PROGRAM DwordToByteArray  //Convert integer value to byte array
VAR_INPUT 
	diValue : DINT;
	Datalenght : DWORD ; 
END_VAR
VAR_IN_OUT
	DataOut:ARRAY[0..255] OF BYTE := (0);
END_VAR
VAR
	
END_VAR


MEMSET(ADR(DataOut), 0, SIZEOF(DataOut));
CASE Datalenght OF
1:
	DataOut[0] := ANY_TO_BYTE(ANY_TO_UDINT(diValue) AND 16#FF); 
2:
	DataOut[0] := ANY_TO_BYTE(ANY_TO_UDINT(diValue) AND 16#FF); 
	DataOut[1] := ANY_TO_BYTE(SHR(ANY_TO_UDINT(diValue) AND 16#FF00,8)); 

ELSE
	DataOut[0] := ANY_TO_BYTE(ANY_TO_UDINT(diValue) AND 16#FF); 
	DataOut[1] := ANY_TO_BYTE(SHR(ANY_TO_UDINT(diValue) AND 16#FF00,8)); 
	DataOut[2] := ANY_TO_BYTE(SHR(ANY_TO_UDINT(diValue) AND 16#FF0000,16)); 
	DataOut[3] := ANY_TO_BYTE(SHR(ANY_TO_UDINT(diValue) AND 16#FF000000,24)); 	
END_CASE;

END_PROGRAM
